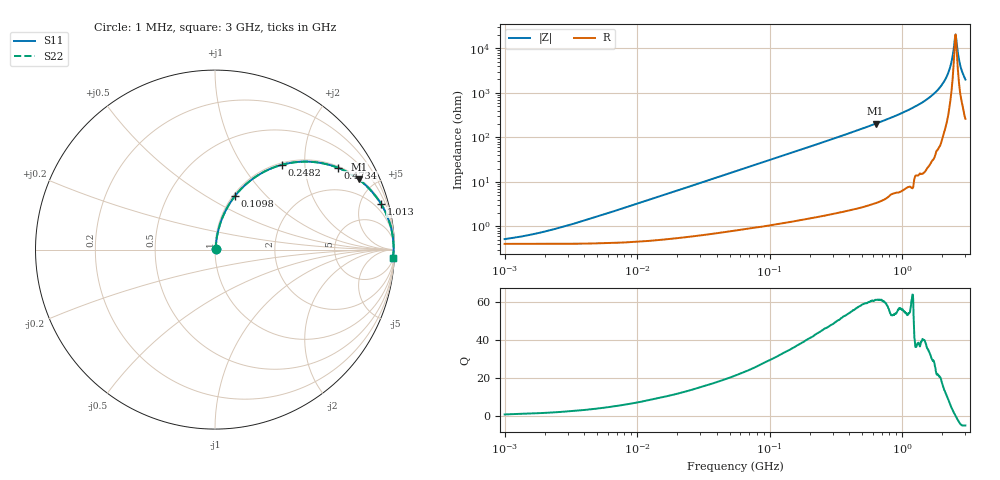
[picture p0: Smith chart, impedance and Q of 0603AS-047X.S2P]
!s-Parameter Generated by FASTRON Sdn. Bhd.
!FASTRON P/N : 0603AS-047X
!Keysight Technologies: E4991B_MY54100416_A.01.15
!Date created: Wed Oct 04 10:58:06 2023
!Version  : Rev01 Wed Oct 04 10:58:06 2023
!Data & Calibration Information:
!Freq	S11	S21	S12	S22
!PortZ  Port1:50+j0  Port2:50+j0
!When reading reference impedance value at option line is always used.
! Remarks : This data is being provided solely for informational purposes.
# Hz S dB R 50
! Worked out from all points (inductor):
!   1601 points, 1 MHz to 3 GHz, reference 50 ohm
!   read as one part in series: L = 51.5 nH near 3.823 MHz
!   highest Q = 61 at 629.6 MHz (marker M1), where L = 51.3 nH
!   self-resonance near 2.518 GHz
!   S11 on the Smith chart (normalised r, x): 1 MHz: 1.01, +0.01; 109.8 MHz: 1.02, +0.68; 248.2 MHz: 1.03, +1.53; 473.4 MHz: 1.05, +2.98; 1.013 GHz: 1.13, +7.22; 3 GHz: 6, -40
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1000000  -45.71 38.6  -0.04 -0.2  -0.04 -0.2  -45.71 38.6
1850562  -42.82 55.6  -0.04 -0.3  -0.04 -0.3  -42.82 55.6
3804036  -37.76 70.9  -0.04 -0.7  -0.04 -0.7  -37.76 70.9
1.447069e7  -26.69 81.3  -0.05 -2.6  -0.05 -2.6  -26.69 81.3
5.477226e7  -15.52 77.7  -0.19 -9.6  -0.19 -9.6  -15.52 77.7
1.098084e8  -9.94 69.6  -0.56 -18.6  -0.56 -18.6  -9.94 69.6
2.083556e8  -5.44 56.3  -1.59 -32.3  -1.59 -32.3  -5.44 56.3
2.482374e8  -4.41 51.7  -2.10 -37.0  -2.10 -37.0  -4.41 51.7
4.733803e8  -1.69 33.6  -5.14 -55.4  -5.14 -55.4  -1.69 33.6
6.296259e8  -1.00 26.0  -7.15 -63.0  -7.15 -63.0  -1.00 26.0
7.925923e8  -0.63 20.5  -9.10 -68.4  -9.10 -68.4  -0.63 20.5
1.01283e9  -0.36 15.4  -11.51 -73.6  -11.51 -73.6  -0.36 15.4
1.503902e9  -0.12 8.3  -16.84 -80.2  -16.84 -80.2  -0.12 8.3
1.950859e9  -0.05 4.1  -22.91 -83.0  -22.91 -83.0  -0.05 4.1
2.244273e9  -0.04 1.9  -29.57 -81.1  -29.57 -81.1  -0.04 1.9
2.347656e9  -0.04 1.2  -33.56 -76.7  -33.56 -76.7  -0.04 1.2
2.468121e9  -0.04 0.4  -41.63 -54.6  -41.63 -54.6  -0.04 0.4
2.51802e9  -0.04 0.1  -46.01 -14.0  -46.01 -14.0  -0.04 0.1
2.594767e9  -0.04 -0.4  -41.06 54.5  -41.06 54.5  -0.04 -0.4
2.700748e9  -0.05 -1.1  -34.20 72.6  -34.20 72.6  -0.05 -1.1
2.797026e9  -0.06 -1.7  -30.61 76.3  -30.61 76.3  -0.06 -1.7
3e9  -0.07 -2.8  -26.06 79.6  -26.06 79.6  -0.07 -2.8
